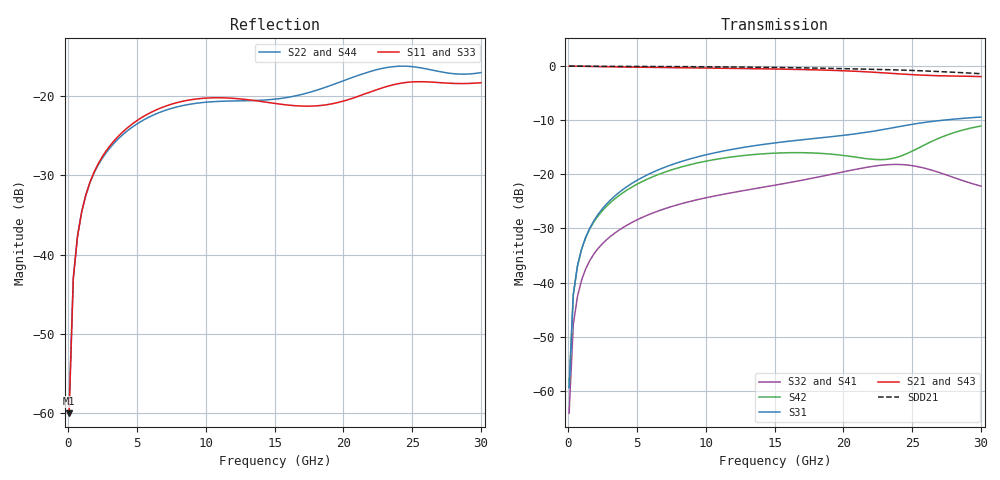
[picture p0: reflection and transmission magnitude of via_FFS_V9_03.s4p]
! Touchstone file written by Full-Wave Solver - Via VX.2.8
! 2021/06/21, 09:49:07
! HyperLynx Advanced Solvers
! Directory: D:/SERDES_Labs/AA_Example/via_FFS_V9_03//via_FFS_V9_03//DUT/
! Project: via_FFS_V9_03  Simulation: DUT
! User: Terry
! Computer: W10ProDesk
! Single-ended  S-parameters
! HL_PORTMAP 1.0
! PORT 1 +(PIN ENTRY.1, S1, S) NAME:S1||ENTRY.1||GND
! PORT 2 +(PIN EXIT.1, S1, S) NAME:S1||EXIT.1||GND
! PORT 3 +(PIN ENTRY.2, S2, S) NAME:S2||ENTRY.2||GND
! PORT 4 +(PIN EXIT.2, S2, S) NAME:S2||EXIT.2||GND
! CONNECT 1, 2;
! CONNECT 3, 4;
! END_HL_PORTMAP
# HZ S RI R 50
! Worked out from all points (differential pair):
!   100 points, 50 MHz to 30 GHz, reference 50 ohm
!   strongest paths, dB at 50 MHz, 7.613 GHz, 15.18 GHz, 22.74 GHz, 30 GHz:
!     S21: 0.0, -0.3, -0.5, -1.2, -1.9
!     S43: 0.0, -0.3, -0.5, -1.2, -1.9
!     S31: -59.4, -18.1, -14.1, -11.8, -9.4
!     S42: -59.4, -19.1, -16.1, -17.3, -11.1
!     S32: -64.2, -25.9, -21.9, -18.3, -22.2
!     S41: -64.2, -25.9, -22.0, -18.4, -22.2
!   taken as a pair (ports 1,3 in; 2,4 out), SDD21 dB: 0.0, -0.1, -0.3, -0.6, -1.4
!   lowest |S11| = -60.0 dB at 50 MHz (marker M1), VSWR 1.00, Z = 50.1 + j0.0556 ohm
!   |S11| at or under -10 dB: start of sweep to end of sweep
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5e7  0.000828 0.000555  0.9988 -0.0102  0.000138 0.00106  -3.26e-05 -0.000615
     0.9988 -0.0102  0.00096 0.000556  4.18e-06 -0.000618  7.87e-05 0.00107
     0.000138 0.00106  4.18e-06 -0.000618  0.000734 0.000741  0.9987 -0.0101
     -3.26e-05 -0.000615  7.87e-05 0.00107  0.9987 -0.0101  0.000869 0.000753
6.550505e8  0.00305 0.0126  0.9897 -0.1276  0.00255 0.0139  -0.00193 -0.00713
            0.9897 -0.1276  0.00399 0.0124  -0.00191 -0.00717  0.00309 0.0139
            0.00255 0.0139  -0.00191 -0.00717  0.00297 0.0125  0.9896 -0.1276
            -0.00193 -0.00713  0.00309 0.0139  0.9896 -0.1276  0.00398 0.0125
2.772727e9  0.0263 0.037  0.8504 -0.5015  0.0305 0.0435  -0.019 -0.0159
            0.8504 -0.5015  0.0338 0.0285  -0.0191 -0.0159  0.034 0.0376
            0.0305 0.0435  -0.0191 -0.0159  0.026 0.037  0.8503 -0.5018
            -0.019 -0.0159  0.034 0.0376  0.8503 -0.5018  0.0341 0.0285
9.125758e9  0.095 0.00845  -0.1473 -0.9514  0.1409 -0.0169  -0.0477 0.0312
            -0.1473 -0.9514  0.0618 -0.0649  -0.048 0.0313  0.1157 -0.0479
            0.1409 -0.0169  -0.048 0.0313  0.0952 0.00984  -0.1478 -0.9512
            -0.0477 0.0312  0.1157 -0.0479  -0.1478 -0.9512  0.0613 -0.0661
1.608384e10  0.0749 -0.0453  -0.9299 -0.0952  0.0572 -0.1942  0.0218 0.0805
             -0.9299 -0.0952  -0.0976 -0.0141  0.022 0.081  -0.0299 -0.1555
             0.0572 -0.1942  0.022 0.081  0.0764 -0.0452  -0.9293 -0.0952
             0.0218 0.0805  -0.0299 -0.1555  -0.9293 -0.0952  -0.0991 -0.0139
2.304192e10  0.0653 -0.0936  -0.2857 0.8159  -0.1965 -0.1725  0.1204 -0.0183
             -0.2857 0.8159  0.1071 0.106  0.1208 -0.0185  -0.1302 -0.0432
             -0.1965 -0.1725  0.1208 -0.0185  0.0654 -0.0946  -0.2864 0.8155
             0.1204 -0.0183  -0.1302 -0.0432  -0.2864 0.8155  0.107 0.1071
3e10  -0.0375 -0.1155  0.6469 0.4709  -0.2676 0.2069  -0.00271 -0.0774
      0.6469 0.4709  0.0685 -0.1228  -0.00419 -0.0776  -0.1855 0.2088
      -0.2676 0.2069  -0.00419 -0.0776  -0.0357 -0.1155  0.6468 0.4711
      -0.00271 -0.0774  -0.1855 0.2088  0.6468 0.4711  0.0671 -0.1238
